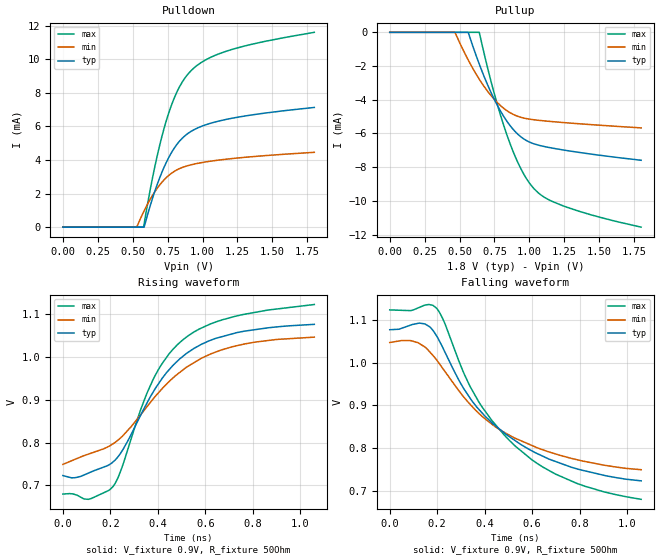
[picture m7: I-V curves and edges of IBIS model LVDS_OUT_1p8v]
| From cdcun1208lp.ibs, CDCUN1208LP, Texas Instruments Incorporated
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[Model]   LVDS_OUT_1p8v
Model_type   Output
Polarity   Non-Inverting
Enable   Active-High
Vmeas = 0.9
Vref = 0.9
Cref = 0pF
Rref = 50
|   typ   min   max
C_comp   6.5137pF   6.0928pF   7.0759pF
[Voltage Range]   1.8   1.7   1.9
[Temperature Range]   27   105   -40
[Pullup Reference]   1.8   1.7   1.9
[Pulldown Reference]   0   0   0
[Power Clamp Reference]   1.8   1.7   1.9
[GND Clamp Reference]   0   0   0
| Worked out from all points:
|   falling waveform, V_fixture 0.9V, R_fixture 50Ohm: 20-80 % time 349ps typ, 365ps min, 339ps max; typ from 1.08 V to 0.723 V
|   rising waveform, V_fixture 0.9V, R_fixture 50Ohm: 20-80 % time 251ps typ, 315ps min, 229ps max; typ from 0.723 V to 1.08 V
[Pulldown]
|   Voltage   I(typ)   I(min)   I(max)
0V        0A         0A         0A
527.8mV   0A         0A         0A
577.4mV   0A         901uA      0A
582mV     0A         978.2uA    198.8uA
658.6mV   2.142mA    2.112mA    3.614mA
735.3mV   3.767mA    2.91mA     6.197mA
775.9mV   4.419mA    3.202mA    7.234mA
816.5mV   4.932mA    3.414mA    8.055mA
902.3mV   5.625mA    3.683mA    9.185mA
1.015V    6.079mA    3.877mA    9.936mA
1.173V    6.428mA    4.054mA    10.49mA
1.8V      7.136mA    4.461mA    11.61mA
[Pullup]
|   Voltage   I(typ)   I(min)   I(max)
0V        0A         0A         0A
464.7mV   0A         0A         0A
559.4mV   0A         -1.602mA   0A
640.6mV   -1.877mA   -2.776mA   0A
739.9mV   -3.829mA   -3.896mA   -3.372mA
834.6mV   -5.224mA   -4.623mA   -5.982mA
884.2mV   -5.762mA   -4.869mA   -7.09mA
929.3mV   -6.134mA   -5.018mA   -7.935mA
1.02V     -6.576mA   -5.174mA   -9.151mA
1.105V    -6.774mA   -5.253mA   -9.779mA
1.236V    -6.972mA   -5.348mA   -10.28mA
1.8V      -7.59mA    -5.669mA   -11.56mA
[Ramp]
R_load = 50
|   typ   min   max
dV/dt_r   0.212275/2.51103e-010  0.178659/3.12285e-010  0.266101/2.28265e-010
dV/dt_f   0.212275/3.48548e-010  0.178659/3.61349e-010  0.266101/3.38506e-010
[Falling Waveform]
V_fixture = 0.9V
V_fixture_min = 0.9V
V_fixture_max = 0.9V
R_fixture = 50Ohm
C_fixture = 0F
|   Time   V(typ)   V(min)   V(max)
0s        1.077V     1.047V     1.123V
127ps     1.092V     1.044V     1.13V
196.6ps   1.063V     1.007V     1.128V
228.8ps   1.029V     982mV      1.096V
299.1ps   951mV      928.3mV    992.8mV
374.5ps   890.9mV    881.5mV    908.5mV
482.8ps   835mV      836.4mV    830mV
597.1ps   793.7mV    806.3mV    773mV
789.2ps   750.9mV    772.4mV    716.8mV
1.059ns   723mV      749.1mV    679.7mV
[Rising Waveform]
V_fixture = 0.9V
V_fixture_min = 0.9V
V_fixture_max = 0.9V
R_fixture = 50Ohm
C_fixture = 0F
|   Time   V(typ)   V(min)   V(max)
0s        723mV      749.1mV    679.7mV
106.8ps   728.5mV    773mV      667.3mV
209.4ps   753.8mV    796.6mV    696.1mV
248.4ps   779.7mV    813.8mV    741mV
327.5ps   864mV      865.1mV    876.8mV
379.3ps   917.3mV    901.5mV    946.6mV
445.7ps   969.4mV    942mV      1.007V
528.3ps   1.012V     979.1mV    1.05V
713.9ps   1.055V     1.024V     1.094V
1.059ns   1.077V     1.047V     1.123V
